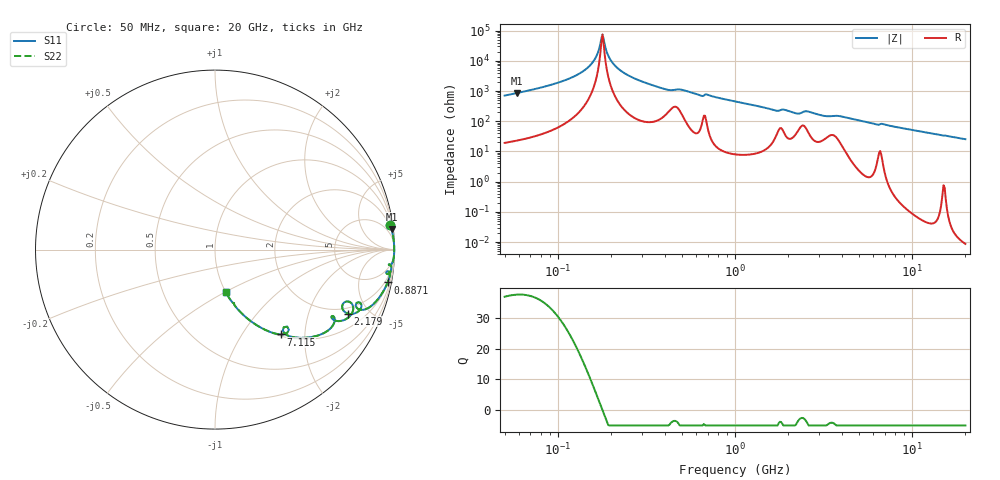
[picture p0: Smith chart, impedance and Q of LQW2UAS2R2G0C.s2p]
!Murata Part Number: LQW2UAS2R2G0C
!These Parameters are Measured in Series Mode Connection
!  o--[Z]--o
!Port1  Port2
!  o-------o
!Freq. Start=50[MHz] Stop=20[GHz], 401[Steps]
# Hz S RI R 50
!Freq.(Hz) S11(Real) S11(Imag) S21(Real) S21(Imag) S12(Real) S12(Imag) S22(Real) S22(Imag)
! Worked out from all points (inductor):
!   401 points, 50 MHz to 20 GHz, reference 50 ohm
!   read as one part in series: L = 2.06 uH near 51.52 MHz
!   highest Q = 37.5 at 58.96 MHz (marker M1), where L = 2.32 uH
!   self-resonance near 176 MHz
!   S11 on the Smith chart (normalised r, x): 50 MHz: 1, +14; 887.1 MHz: 1, -10; 2.179 GHz: 1.68, -3.65; 7.115 GHz: 1.03, -1.51; 20 GHz: 1.00, -0.51
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5e7  0.9768 0.1376  0.0232 -0.1376  0.0232 -0.1376  0.9768 0.1376
5.895582e7  0.9837 0.1139  0.0163 -0.1139  0.0163 -0.1139  0.9837 0.1139
9.958798e7  0.9954 0.0531  0.00458 -0.0531  0.00458 -0.0531  0.9954 0.0531
1.364002e8  0.998 0.0236  0.00197 -0.0236  0.00197 -0.0236  0.998 0.0236
1.584406e8  0.9985 0.0104  0.00146 -0.0104  0.00146 -0.0104  0.9985 0.0104
1.657227e8  0.9986 0.00645  0.00138 -0.00645  0.00138 -0.00645  0.9986 0.00645
1.759554e8  0.9987 0.00122  0.00134 -0.00122  0.00134 -0.00122  0.9987 0.00122
1.786108e8  0.9987 -8.28e-05  0.00134 8.28e-05  0.00134 8.28e-05  0.9987 -8.28e-05
1.813063e8  0.9987 -0.00139  0.00134 0.00139  0.00134 0.00139  0.9987 -0.00139
1.983553e8  0.9985 -0.00928  0.00145 0.00928  0.00145 0.00928  0.9985 -0.00928
2.202824e8  0.9982 -0.0186  0.0018 0.0186  0.0018 0.0186  0.9982 -0.0186
2.676374e8  0.9968 -0.037  0.00321 0.037  0.00321 0.037  0.9968 -0.037
3.721004e8  0.9882 -0.0738  0.0118 0.0738  0.0118 0.0738  0.9882 -0.0738
4.946044e8  0.9775 -0.0849  0.0225 0.0849  0.0225 0.0849  0.9775 -0.0849
8.870719e8  0.9618 -0.1828  0.0382 0.1828  0.0382 0.1828  0.9618 -0.1828
1e9  0.9502 -0.209  0.0498 0.209  0.0498 0.209  0.9502 -0.209
2.179053e9  0.739 -0.3561  0.261 0.3561  0.261 0.3561  0.739 -0.3561
2.419936e9  0.7354 -0.2884  0.2646 0.2884  0.2646 0.2884  0.7354 -0.2884
2.728004e9  0.7562 -0.3651  0.2438 0.3651  0.2438 0.3651  0.7562 -0.3651
7.114996e9  0.367 -0.473  0.633 0.473  0.633 0.473  0.367 -0.473
7.442007e9  0.3382 -0.4685  0.6618 0.4685  0.6618 0.4685  0.3382 -0.4685
2e10  0.0606 -0.2384  0.9394 0.2384  0.9394 0.2384  0.0606 -0.2384
